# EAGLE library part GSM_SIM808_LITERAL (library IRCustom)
SIM808 GSM Module
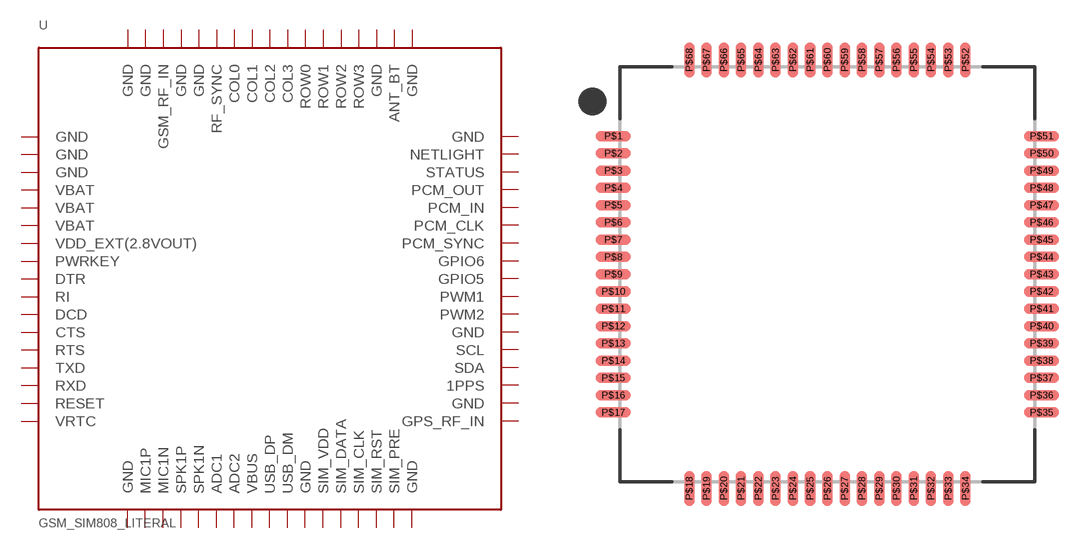
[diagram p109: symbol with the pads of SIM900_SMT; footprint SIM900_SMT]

Designator prefix U

## GSM_SIM808_LITERAL  [SIM900_SMT]
P$1  GND  pwr
P$2  GND  pwr
P$3  GND  pwr
P$4  VBAT  pwr
P$5  VBAT  pwr
P$6  VBAT  pwr
P$7  VDD_EXT(2.8VOUT)  pwr
P$8  PWRKEY  in
P$9  DTR  in
P$10  RI  out
P$11  DCD  out
P$12  CTS  out
P$13  RTS  in
P$14  TXD  out
P$15  RXD  in
P$16  RESET  in
P$17  VRTC  pwr
P$18  GND  pwr
P$19  MIC1P  in
P$20  MIC1N  in
P$21  SPK1P  out
P$22  SPK1N  out
P$23  ADC1  in
P$24  ADC2  in
P$25  VBUS  pwr
P$26  USB_DP
P$27  USB_DM
P$28  GND  pwr
P$29  SIM_VDD  pwr
P$30  SIM_DATA
P$31  SIM_CLK  out
P$32  SIM_RST  out
P$33  SIM_PRE  in
P$34  GND  pwr
P$35  GPS_RF_IN
P$36  GND  pwr
P$37  1PPS  in
P$38  SDA
P$39  SCL  out
P$40  GND  pwr
P$41  PWM2  out
P$42  PWM1  out
P$43  GPIO5
P$44  GPIO6
P$45  PCM_SYNC  out
P$46  PCM_CLK  in
P$47  PCM_IN  in
P$48  PCM_OUT  out
P$49  STATUS  out
P$50  NETLIGHT  out
P$51  GND  pwr
P$52  GND  pwr
P$53  ANT_BT
P$54  GND  pwr
P$55  ROW3  out
P$56  ROW2  out
P$57  ROW1  out
P$58  ROW0  out
P$59  COL3  in
P$60  COL2  in
P$61  COL1  in
P$62  COL0  in
P$63  RF_SYNC  out
P$64  GND  pwr
P$65  GND  pwr
P$66  GSM_RF_IN  in
P$67  GND  pwr
P$68  GND  pwr

## Footprint SIM900_SMT (pad centres in mm)
smd 2 x 0.6: P$1 -12.4,8; P$2 -12.4,7; P$3 -12.4,6; P$4 -12.4,5; P$5 -12.4,4; P$6 -12.4,3; P$7 -12.4,2; P$8 -12.4,1; P$9 -12.4,0; P$10 -12.4,-1; P$11 -12.4,-2; P$12 -12.4,-3; P$13 -12.4,-4; P$14 -12.4,-5; P$15 -12.4,-6; P$16 -12.4,-7; P$17 -12.4,-8; P$35 12.4,-8; P$36 12.4,-7; P$37 12.4,-6; P$38 12.4,-5; P$39 12.4,-4; P$40 12.4,-3; P$41 12.4,-2; P$42 12.4,-1; P$43 12.4,0; P$44 12.4,1; P$45 12.4,2; P$46 12.4,3; P$47 12.4,4; P$48 12.4,5; P$49 12.4,6; P$50 12.4,7; P$51 12.4,8
smd 0.6 x 2: P$18 -8,-12.4; P$19 -7,-12.4; P$20 -6,-12.4; P$21 -5,-12.4; P$22 -4,-12.4; P$23 -3,-12.4; P$24 -2,-12.4; P$25 -1,-12.4; P$26 0,-12.4; P$27 1,-12.4; P$28 2,-12.4; P$29 3,-12.4; P$30 4,-12.4; P$31 5,-12.4; P$32 6,-12.4; P$33 7,-12.4; P$34 8,-12.4; P$52 8,12.4; P$53 7,12.4; P$54 6,12.4; P$55 5,12.4; P$56 4,12.4; P$57 3,12.4; P$58 2,12.4; P$59 1,12.4; P$60 0,12.4; P$61 -1,12.4; P$62 -2,12.4; P$63 -3,12.4; P$64 -4,12.4; P$65 -5,12.4; P$66 -6,12.4; P$67 -7,12.4; P$68 -8,12.4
